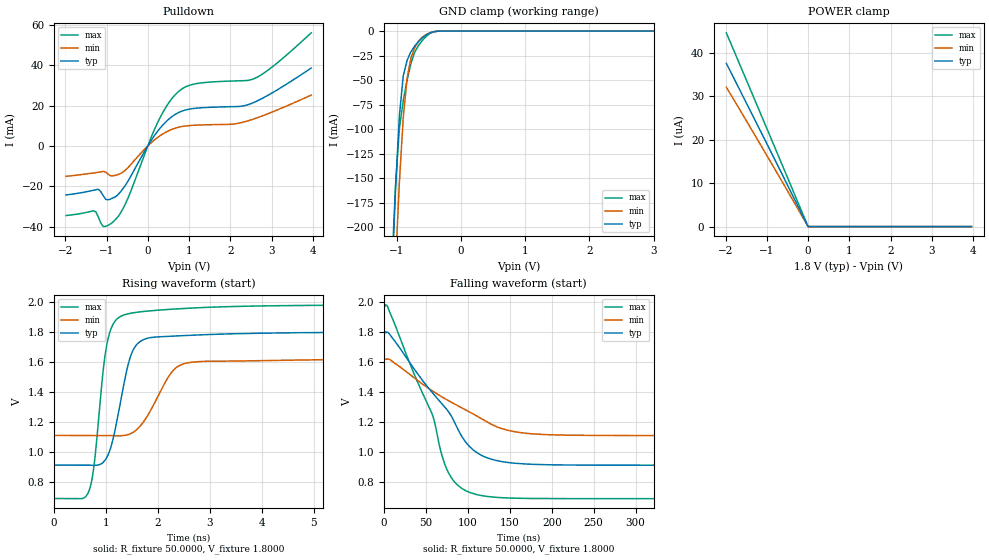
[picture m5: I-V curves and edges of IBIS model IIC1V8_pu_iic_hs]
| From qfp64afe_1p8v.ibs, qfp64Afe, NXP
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[Model] IIC1V8_pu_iic_hs
|   Model IIC1V8_pu_iic_hs
| This model was characterised for following simulation conditions:
| External (pad) voltage:
|   - Typ: 1.8V,   - Min: 1.62V,   - Max: 1.98V
| Library cells for typ/min/max conditions are connected as defined below:
|  IO - External Pad
|  A - Core Input
|  EN - Output Buffer Enable
|  BOOST - vdde
|  ECS - gnd
|  EGP - gnd
|  ENZI - vdd
|  EPD - gnd
|  EPUN - gnd
|  ZI - NC
|  ZIF - NC
|  gnd - gnd
|  gnde - gnde
|  vdd - vdd
|  vdde - vdde
| All other pins connected to ground
Model_type I/O_open_drain
Polarity   Non-Inverting
Enable   Active-Low
Vinl =   0.5400V
Vinh =   1.2600V
Vmeas =  0.9000V
Cref =   0.0F
Rref =   1000.000
Vref =   1.8000V
C_comp   3.6102pF   3.4624pF   3.7516pF
|C_comp_pullup   0.9283pF   0.9069pF   0.9343pF
|C_comp_pulldown   2.3311pF   2.4844pF   2.1853pF
[Model Spec]
| variable   typ   min   max
Vinh   0.5400V   0.4860V   0.5940V
Vinl   1.2600V   1.1340V   1.3860V
Vmeas   0.9000V   0.8100V   0.9900V
Vref   1.8000V   1.6200V   1.9800V
Cref   0.0F   0.0F   0.0F
Rref   1.0000k   1.0000k   1.0000k
[Temperature Range]   25.0000   0.1250k   -40.0000
[Voltage Range]   1.8000V   1.6200V   1.9800V
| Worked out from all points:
|   slope of the pulldown table from 0 to 0.27 V, typ, clamps not added: 33.4 ohm
|   GND clamp passes 1 mA (typ) near -0.44 V on its own axis
|   rising waveform, R_fixture 50.0000, V_fixture 1.8000: 20-80 % time 320ps typ, 490ps min, 236ps max; typ from 0.912 V to 1.8 V
|   falling waveform, R_fixture 50.0000, V_fixture 1.8000: 20-80 % time 67ns typ, 88.7ns min, 49ns max; typ from 1.8 V to 0.912 V
[Pulldown]
|Voltage   I(typ)   I(min)   I(max)
-1.98V    -24.22mA   -15.04mA   -34.42mA
-1.32V    -21.94mA   -13.4mA    -32.06mA
-1.2V     -21.45mA   -13.05mA   -35.06mA
-1.08V    -24.63mA   -12.6mA    -39.9mA
-900mV    -26.23mA   -14.78mA   -38.53mA
-540mV    -19.33mA   -11.9mA    -28.53mA
300mV     8.856mA    5.096mA    14.12mA
720mV     16.26mA    9.117mA    26.48mA
1.14V     18.6mA     10.26mA    30.69mA
2.1V      19.45mA    10.89mA    32.16mA
2.58V     21.61mA    13.43mA    33.34mA
3.96V     38.54mA    25.17mA    55.97mA
[GND_clamp]
|Voltage   I(typ)   I(min)   I(max)
-1.98V    -2.104A    -2.075A    -2.136A
-1.08V    -259.3mA   -333mA     -247mA
-1.02V    -161.8mA   -238.7mA   -157.2mA
-960mV    -86.78mA   -154.8mA   -99.51mA
-900mV    -45.99mA   -88.85mA   -71.1mA
-840mV    -29.94mA   -48.03mA   -50.31mA
-780mV    -21.2mA    -27.67mA   -33.04mA
-720mV    -15.2mA    -16.91mA   -21.32mA
-660mV    -10.61mA   -10.27mA   -14.61mA
-540mV    -3.83mA    -3.432mA   -5.346mA
-300mV    -56.31uA   -67.68uA   -68.13uA
3.96V     0A         0A         0A
[POWER_clamp]
|Voltage   I(typ)   I(min)   I(max)
-1.98V    37.59uA    32.11uA    44.63uA
-960mV    18.36uA    15.76uA    21.73uA
0V        104.7pA    4.893nA    11.38pA
3.96V     0A         0A         0A
[Ramp]
| variable   typ   min   max
dV/dt_r  0.5330/0.3204n   0.3064/0.4905n   0.7749/0.2364n
dV/dt_f  0.5329/66.9544n   0.3063/88.6897n   0.7748/48.9915n
R_load = 50.0000
[Rising Waveform]
R_fixture= 50.0000
V_fixture= 1.8000
V_fixture_min= 1.6200
V_fixture_max= 1.9800
|time   V(typ)   V(min)   V(max)
0s        911.7mV    1.109V     688.6mV
683.6ps   910.9mV    1.109V     746.6mV
780.7ps   909.8mV    1.109V     929.5mV
1.004ns   954mV      1.109V     1.686V
1.256ns   1.282V     1.107V     1.897V
1.505ns   1.663V     1.126V     1.926V
1.78ns    1.756V     1.228V     1.938V
2.495ns   1.775V     1.587V     1.956V
5.696ns   1.797V     1.616V     1.978V
1us       1.8V       1.62V      1.98V
[Falling Waveform]
R_fixture= 50.0000
V_fixture= 1.8000
V_fixture_min= 1.6200
V_fixture_max= 1.9800
|time   V(typ)   V(min)   V(max)
0s        1.8V       1.62V      1.98V
4.153ns   1.8V       1.621V     1.974V
56.84ns   1.402V     1.411V     1.262V
69.16ns   1.323V     1.368V     975.9mV
77.26ns   1.267V     1.342V     857.9mV
94.24ns   1.092V     1.291V     752.2mV
111.1ns   994.8mV    1.239V     715.3mV
146.8ns   931mV      1.146V     693.6mV
207.1ns   914.2mV    1.114V     689.1mV
1us       911.8mV    1.109V     688.6mV
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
